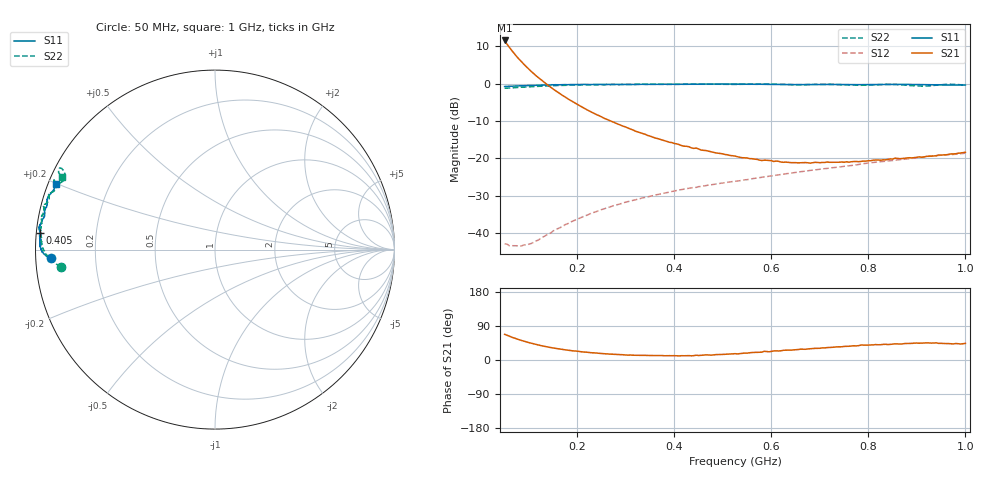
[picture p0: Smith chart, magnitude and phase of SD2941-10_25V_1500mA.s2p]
!Agilent Technologies,E8358A,US42080673,A.04.86
!Agilent E8358A: A.04.86
!Date: Friday, June 09, 2006 14:45:18
!Correction: S11(Full 2 Port SOLT,1,2) S21(Full 2 Port SOLT,1,2) S12(Full 2 Port SOLT,1,2) S22(Full 2 Port SOLT,1,2)
!S2P File: Measurements: S11, S21, S12, S22:
# Hz S  MA  R 50
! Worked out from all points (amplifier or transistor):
!   191 points, 50 MHz to 1 GHz, reference 50 ohm
!   highest |S21| = 11.5 dB at 50 MHz (marker M1)
!   |S21| within 3 dB of that: start of sweep to 66.76 MHz
!   unconditionally stable (mu >= 1): 751.2 MHz to 816.8 MHz; 874.6 MHz to 958.1 MHz; 988.7 MHz to end of sweep
!   at 205 MHz: K = 0.46, MSG = 15.0 dB, |S12| = -36.0 dB
!   at 525 MHz: K = 0.49, MSG = 3.4 dB, |S12| = -26.1 dB
!   at 1 GHz: K = 1.10, MAG = -1.8 dB, |S12| = -18.6 dB
!   S11 on the Smith chart (normalised r, x): 50 MHz: 0.05, -0.03; 405 MHz: 0.01, +0.05; 1 GHz: 0.02, +0.20
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5e7  0.9132 -177.0  3.77 67.8  0.00724 14.1  0.8659 -173.6
5.5e7  0.9193 -177.2  3.362 65.4  0.007157 16.8  0.871 -173.8
6e7  0.9205 -177.2  3.041 62.8  0.0068 19.7  0.8725 -174.1
6.5e7  0.9226 -177.2  2.755 60.0  0.006824 21.4  0.8775 -174.2
7.5e7  0.928 -177.4  2.297 55.6  0.006813 27.5  0.8857 -174.6
9e7  0.9388 -177.7  1.804 49.4  0.006986 38.7  0.8976 -175.3
1.05e8  0.9451 -178.2  1.45 44.2  0.007316 49.0  0.9103 -176.0
1.25e8  0.9536 -178.6  1.123 38.0  0.008604 60.0  0.9234 -176.9
1.5e8  0.9636 -179.3  0.8461 31.7  0.01073 68.8  0.9391 -178.1
1.75e8  0.9689 -179.9  0.6609 26.8  0.01305 73.5  0.9486 -179.2
2.1e8  0.9725 179.3  0.4842 21.4  0.01648 76.4  0.9602 179.3
2.8e8  0.9753 177.3  0.2944 14.8  0.02386 78.5  0.9688 176.3
3.7e8  0.9797 175.6  0.1806 11.8  0.03336 77.6  0.9763 172.9
4.05e8  0.9808 174.5  0.1565 11.1  0.03742 76.5  0.9753 171.4
5.25e8  0.9841 172.1  0.1074 16.7  0.04936 73.6  0.9754 167.5
5.8e8  0.9786 171.1  0.09383 20.6  0.05576 72.5  0.9839 165.7
6.85e8  0.9711 168.1  0.08748 30.0  0.06972 69.5  0.9729 162.0
8.45e8  0.9755 163.6  0.09835 41.3  0.09312 64.8  0.9766 156.8
8.9e8  0.9755 162.4  0.1017 43.9  0.1006 62.9  0.9378 156.6
9.25e8  0.9677 161.3  0.1072 45.1  0.1071 62.5  0.9317 153.5
9.6e8  0.9586 159.6  0.1118 43.3  0.1116 60.4  0.9762 152.2
1e9  0.9568 157.5  0.121 43.8  0.1178 56.9  0.9439 154.7
